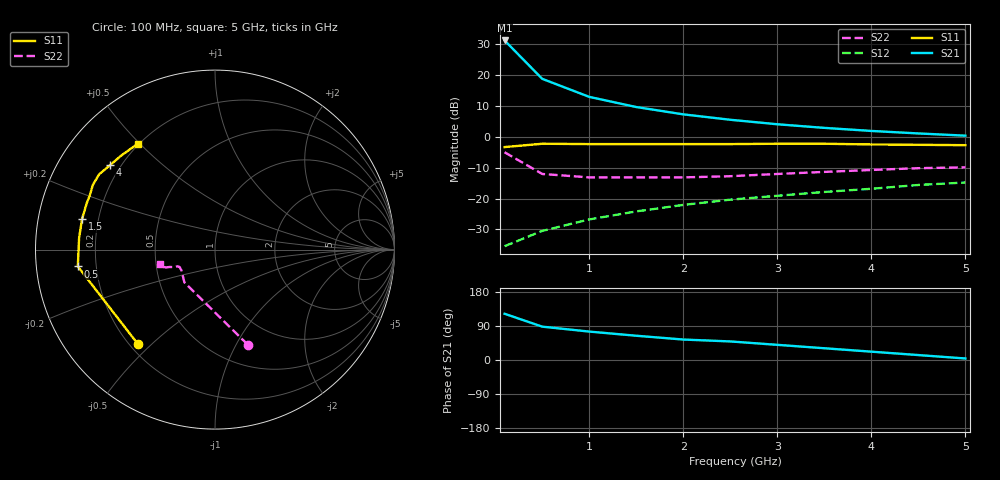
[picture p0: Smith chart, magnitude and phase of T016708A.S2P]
!AT-01670
!S-PARAMETERS at Vce=8V  Ic=35mA.  LAST UPDATED 07-21-92
!OBSOLETED Feb 1994 - nearest replacement: AT-42070
# ghz s ma r 50
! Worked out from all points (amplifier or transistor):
!   11 points, 100 MHz to 5 GHz, reference 50 ohm
!   highest |S21| = 31.1 dB at 100 MHz (marker M1)
!   |S21| within 3 dB of that: start of sweep to 196.7 MHz
!   unconditionally stable (mu >= 1): 772.2 MHz to end of sweep
!   at 500 MHz: K = 0.82, MSG = 24.6 dB, |S12| = -30.5 dB
!   at 2.5 GHz: K = 1.25, MAG = 9.9 dB, |S12| = -20.4 dB
!   at 5 GHz: K = 1.17, MAG = 5.1 dB, |S12| = -14.8 dB
!   S11 on the Smith chart (normalised r, x): 100 MHz: 0.23, -0.46; 500 MHz: 0.13, -0.06; 1.5 GHz: 0.14, +0.11; 4 GHz: 0.16, +0.35; 5 GHz: 0.20, +0.49
0.1  0.68 -129.0  36.01 122.0  0.017 47.0  0.56 -71.0
0.5  0.77 -173.0  8.63 88.0  0.03 42.0  0.25 -133.0
1  0.76 175.0  4.41 75.0  0.046 55.0  0.22 -148.0
1.5  0.76 167.0  3.02 64.0  0.062 54.0  0.22 -153.0
2  0.76 160.0  2.3 54.0  0.079 55.0  0.22 -154.0
2.5  0.76 157.0  1.88 49.0  0.096 58.0  0.23 -156.0
3  0.77 152.0  1.59 40.0  0.111 55.0  0.25 -157.0
3.5  0.77 147.0  1.39 31.0  0.128 50.0  0.27 -159.0
4  0.75 141.0  1.24 22.0  0.144 49.0  0.29 -160.0
4.5  0.74 135.0  1.13 13.0  0.166 44.0  0.31 -162.0
5  0.73 126.0  1.04 4.0  0.182 39.0  0.32 -165.0
